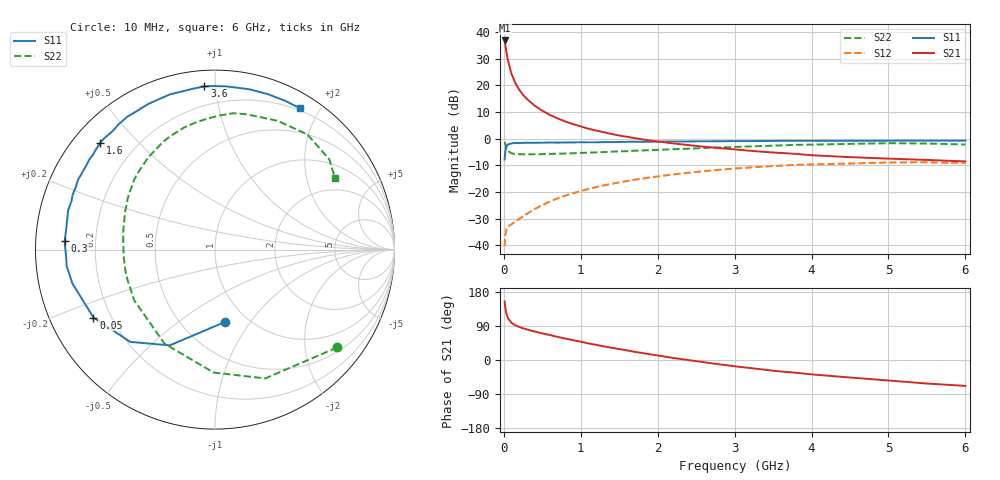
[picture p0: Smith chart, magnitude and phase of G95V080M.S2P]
! SIEMENS Small Signal Semiconductors
! BFG235
! Si NPN RF Bipolar Junction Transistor in SOT223
! VCE = 5 V  IC = 80 mA
! Common Emitter S-Parameters:  July  1994
# GHz  S  MA  R  50
!  f  S11  S21  S12  S22
! GHz  MAG  ANG  MAG  ANG  MAG  ANG  MAG  ANG
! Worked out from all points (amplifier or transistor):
!   40 points, 10 MHz to 6 GHz, reference 50 ohm
!   highest |S21| = 36.8 dB at 10 MHz (marker M1)
!   |S21| within 3 dB of that: start of sweep to 26.14 MHz
!   unconditionally stable (mu >= 1): 482.4 MHz to 1.443 GHz
!   at 200 MHz: K = 0.75, MSG = 24.2 dB, |S12| = -30.0 dB
!   at 1.5 GHz: K = 0.99, MSG = 8.8 dB, |S12| = -16.4 dB
!   at 6 GHz: K = 0.90, MSG = 0.3 dB, |S12| = -9.1 dB
!   S11 on the Smith chart (normalised r, x): 10 MHz: 0.79, -0.76; 50 MHz: 0.13, -0.26; 300 MHz: 0.09, +0.03; 1.6 GHz: 0.08, +0.39; 3.6 GHz: 0.09, +0.93; 6 GHz: 0.17, +1.76
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0.01  0.4077 -82.5  69.06 154.9  0.0097 66.2  0.8721 -38.7
0.02  0.5901 -115.3  55.86 136.7  0.0156 51.2  0.7702 -68.7
0.03  0.6984 -132.6  44.97 124.7  0.019 42.7  0.6847 -90.7
0.05  0.7756 -150.8  30.5 111.3  0.0222 34.6  0.5946 -118.3
0.1  0.817 -166.7  16.31 98.1  0.0251 33.9  0.5314 -147.8
0.15  0.8316 -173.8  10.98 91.5  0.0281 38.9  0.516 -160.3
0.2  0.8303 -177.5  8.229 87.3  0.0315 42.9  0.5128 -167.3
0.25  0.8353 179.0  6.628 83.6  0.0351 46.4  0.5096 -172.0
0.3  0.8385 176.7  5.54 80.8  0.0392 49.4  0.5101 -175.9
0.4  0.8371 172.0  4.166 75.1  0.048 53.5  0.5104 178.8
0.5  0.8407 168.2  3.328 70.2  0.0571 55.1  0.5139 174.5
0.6  0.847 165.1  2.779 65.8  0.0667 55.7  0.5184 170.6
0.7  0.844 161.5  2.393 60.9  0.0763 55.7  0.5233 167.2
0.8  0.8501 158.8  2.096 56.6  0.0859 55.0  0.5265 164.1
1.1  0.8556 149.5  1.536 43.7  0.1144 51.1  0.5474 155.3
1.6  0.8737 137.1  1.085 25.4  0.1609 42.0  0.5837 141.8
2.2  0.887 123.5  0.816 5.5  0.2133 29.2  0.6345 125.8
3.2  0.9 101.9  0.594 -21.2  0.2889 6.0  0.7151 99.1
3.6  0.9115 93.7  0.54 -30.4  0.3124 -4.1  0.7486 87.7
4.5  0.9137 77.8  0.451 -46.2  0.3428 -24.3  0.7977 64.1
5.5  0.9164 64.6  0.4 -62.1  0.3606 -46.5  0.8114 38.3
6  0.9192 58.8  0.375 -68.3  0.3502 -54.8  0.7783 30.8
